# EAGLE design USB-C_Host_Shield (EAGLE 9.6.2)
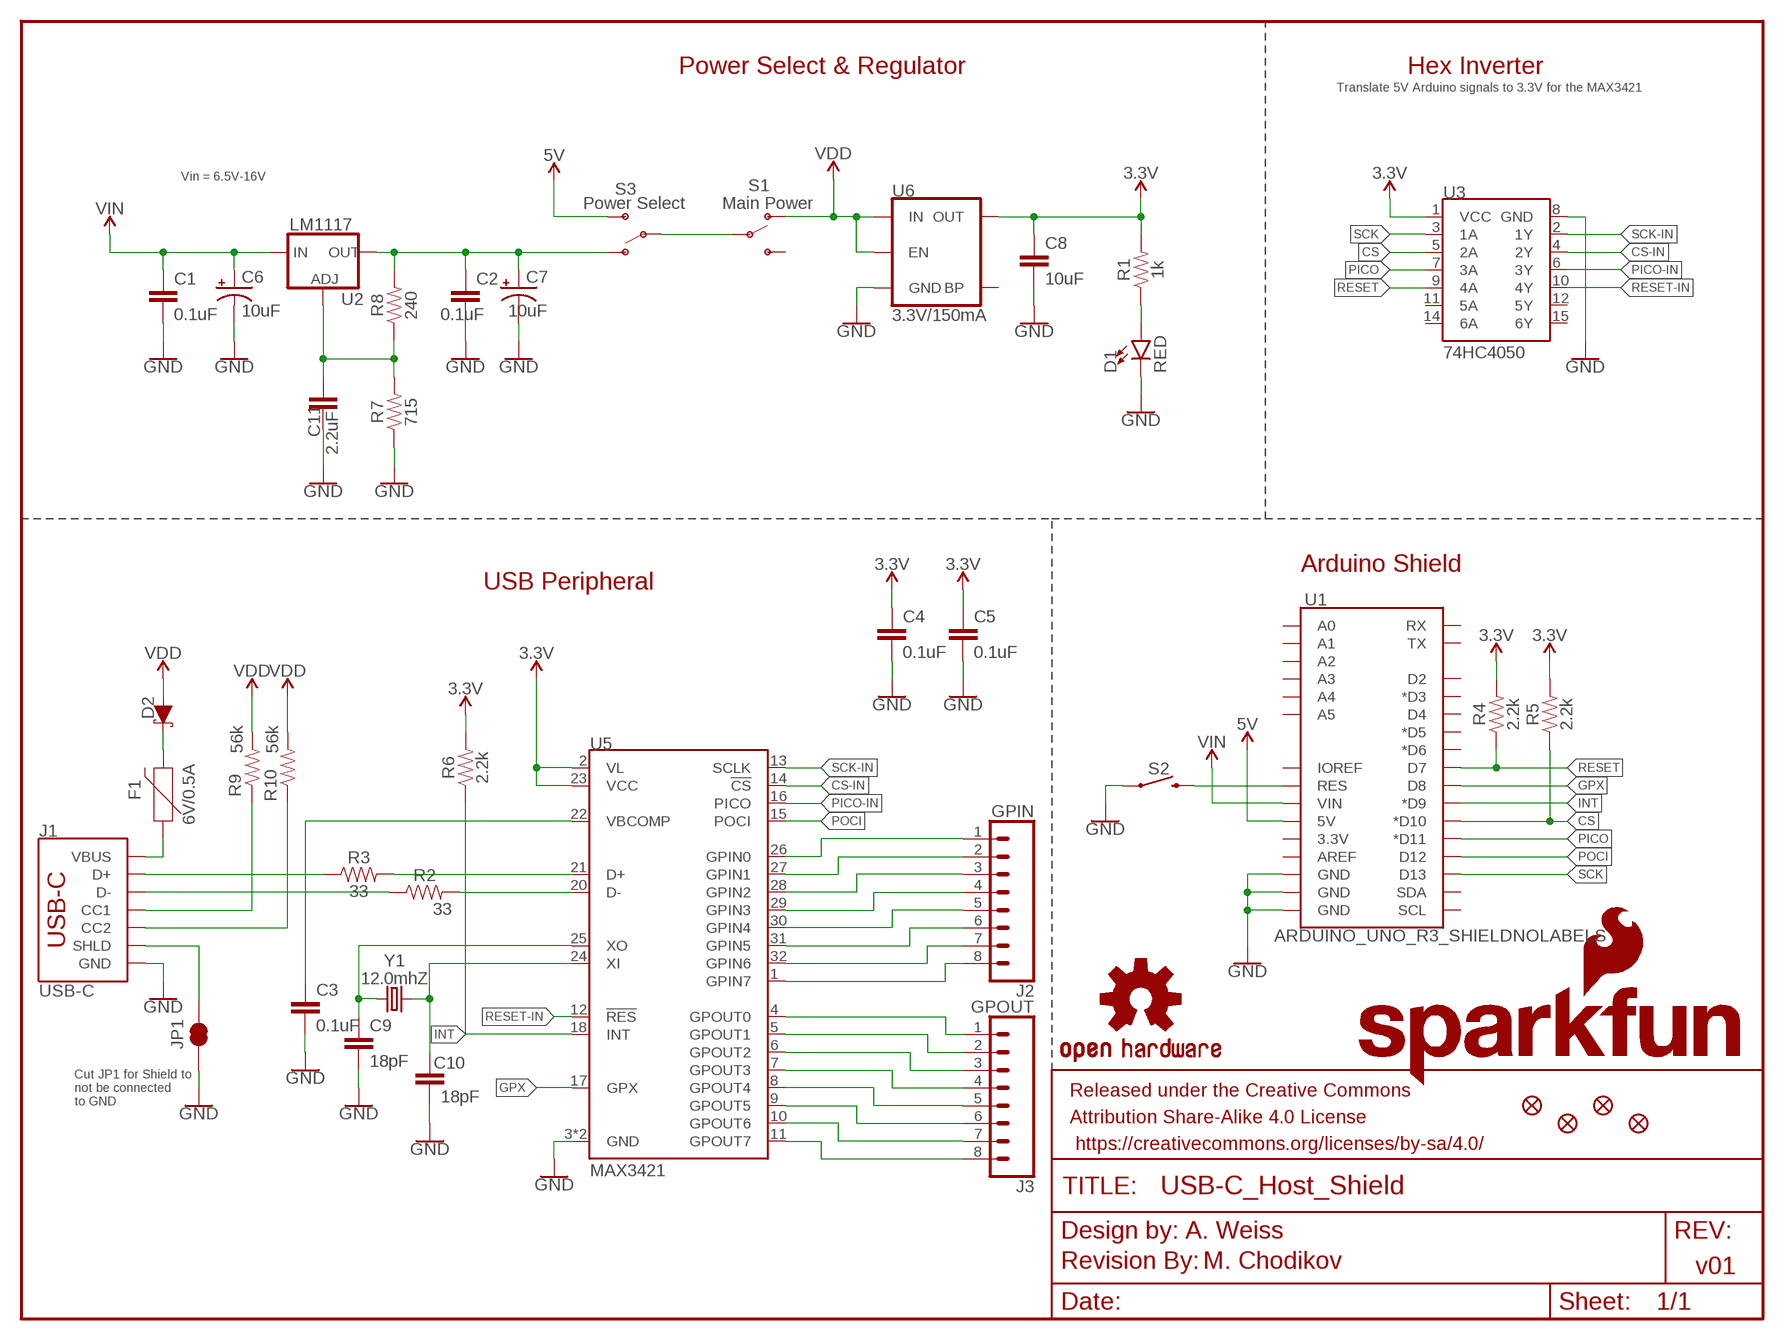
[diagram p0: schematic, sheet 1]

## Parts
C1  0.1uF  0.1UF-0603-25V-(+80/-20%)  [0603]
C2  0.1uF  0.1UF-0603-25V-(+80/-20%)  [0603]
C3  0.1uF  0.1UF-0603-25V-(+80/-20%)  [0603]
C4  0.1uF  0.1UF-0603-25V-(+80/-20%)  [0603]
C5  0.1uF  0.1UF-0603-25V-(+80/-20%)  [0603]
C6  10uF  10UF-POLAR-EIA3216-16V-10%(TANT)  [EIA3216]
C7  10uF  10UF-POLAR-EIA3216-16V-10%(TANT)  [EIA3216]
C8  10uF  10UF-0603-6.3V-20%  [0603]
C9  18pF  18PF-0603-50V-5%  [0603]
C10  18pF  18PF-0603-50V-5%  [0603]
C11  2.2uF  2.2UF-0603-10V-20%  [0603]
D1  RED  LED-RED0603  [LED-0603]
D2  1A/15V/220mV  DIODE-SCHOTTKY-LSM115JE3  [DO-214BA]
F1  6V/0.5A  PPTC_6V500MA-2  [1206]
FD1  FIDUCIALUFIDUCIAL  [FIDUCIAL-MICRO]
FD2  FIDUCIALUFIDUCIAL  [FIDUCIAL-MICRO]
FD3  FIDUCIALUFIDUCIAL  [FIDUCIAL-MICRO]
FD4  FIDUCIALUFIDUCIAL  [FIDUCIAL-MICRO]
FRAME1  FRAME-LETTER  [CREATIVE_COMMONS]
J1  USB-C  USB_C_2-LAYER_PADS  [USB-C-16P-2LAYER-PADS]
J2  GPIN  CONN_08"  [1X08]
J3  GPOUT  CONN_08"  [1X08]
JP1  JUMPER-SMT_2_NC_TRACE_SILK  [SMT-JUMPER_2_NC_TRACE_SILK]
LOGO1  OSHW-LOGOM  [OSHW-LOGO-M]
LOGO2  SFE_LOGO_NAME_FLAME.1_INCH  [SFE_LOGO_NAME_FLAME_.1]
LOGO3  SFE_LOGO_NAME_FLAME.2_INCH  [SFE_LOGO_NAME_FLAME_.2]
LOGO7  REVISION  [REVISION]
R1  1k  1KOHM-0603-1/10W-1%  [0603]
R2  33  33OHM-0603-1/10W-1%  [0603]
R3  33  33OHM-0603-1/10W-1%  [0603]
R4  2.2k  2.2KOHM-0603-1/10W-1%  [0603]
R5  2.2k  2.2KOHM-0603-1/10W-1%  [0603]
R6  2.2k  2.2KOHM-0603-1/10W-1%  [0603]
R7  715  715OHM-0603-1/10W-1%  [0603]
R8  240  240OHM-0603-1/10W-1%  [0603]
R9  56k  56KOHM  [0603]
R10  56k  56KOHM  [0603]
S1  Main Power  SWITCH-SPDT-SMD-AYZ0202  [SWITCH_DPDT_SMD_AYZ0202]
S2  MOMENTARY-SWITCH-SPST-SMD-5.2MM-TALL  [TACTILE_SWITCH_SMD_5.2MM]
S3  Power Select  SWITCH-SPDT-SMD-AYZ0202  [SWITCH_DPDT_SMD_AYZ0202]
U1  ARDUINO_UNO_R3_SHIELDNOLABELS  [UNO_R3_SHIELD_NOLABELS]
U2  LM1117  V_REG_LM1117SOT223  [SOT223]
U3  74HC4050  HEX_CONVERTER  [SO16]
U5  MAX3421  [TQFP32]
U6  3.3V/150mA  V_REG_MIC52053.3V  [SOT23-5]
Y1  12.0mhZ  CRYSTAL-12MHZ  [CRYSTAL-SMD-2X2.5MM]

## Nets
3.3V: C4.1 C5.1 C8.1 R1.2 R4.2 R5.2 R6.2 U3.1(VCC) U5.2(VL) U5.23(VCC) U6.5(OUT)
5V: S3.3(S) U1.5V
CC1: J1.A5(CC1) R9.1
CC2: J1.B5(CC2) R10.1
CS: R5.1 U1.D10(*D10) U3.5(2A)
CS-IN: U3.4(2Y) U5.14(!CS)
D_N [diff pairs]: J1.A7(D-) J1.B7(D-) R2.1
D_P [diff pairs]: J1.A6(D+) J1.B6(D+) R3.1
GND: C1.2 C2.2 C3.2 C4.2 C5.2 C6.- C7.- C8.2 C9.2 C10.2 C11.2 D1.C J1.GND J1.GND2(GND) JP1.1 R7.1 S2.1 U1.GND@0(GND) U1.GND@1(GND) U1.GND@2(GND) U3.8(GND) U5.3(GND) U5.19(GND) U6.2(GND)
GPIN0: J2.1 U5.26(GPIN0)
GPIN1: J2.2 U5.27(GPIN1)
GPIN2: J2.3 U5.28(GPIN2)
GPIN3: J2.4 U5.29(GPIN3)
GPIN4: J2.5 U5.30(GPIN4)
GPIN5: J2.6 U5.31(GPIN5)
GPIN6: J2.7 U5.32(GPIN6)
GPIN7: J2.8 U5.1(GPIN7)
GPOUT0: J3.1 U5.4(GPOUT0)
GPOUT1: J3.2 U5.5(GPOUT1)
GPOUT2: J3.3 U5.6(GPOUT2)
GPOUT3: J3.4 U5.7(GPOUT3)
GPOUT4: J3.5 U5.8(GPOUT4)
GPOUT5: J3.6 U5.9(GPOUT5)
GPOUT6: J3.7 U5.10(GPOUT6)
GPOUT7: J3.8 U5.11(GPOUT7)
GPX: U1.D8 U5.17(GPX)
INT: R6.1 U1.D9(*D9) U5.18(INT)
MAX_D_N: R2.2 U5.20(D-)
MAX_D_P: R3.2 U5.21(D+)
N$1: S2.3 U1.RES
N$2: S1.2(P) S3.2(P)
N$4: C11.1 R7.2 R8.1 U2.1(ADJ)
N$5: D2.C F1.2
N$6: C2.1 C7.+ R8.2 S3.1(O) U2.2(OUT) U2.4(OUT)
N$7: D1.A R1.1
N$8: J1.SHLD1(SHLD) J1.SHLD2(SHLD) J1.SHLD3(SHLD) J1.SHLD4(SHLD) JP1.2
PICO: U1.D11(*D11) U3.7(3A)
PICO-IN: U3.6(3Y) U5.16(PICO)
POCI: U1.D12 U5.15(POCI)
RESET: R4.1 U1.D7 U3.9(4A)
RESET-IN: U3.10(4Y) U5.12(!RES)
SCK: U1.D13 U3.3(1A)
SCK-IN: U3.2(1Y) U5.13(SCLK)
VBCOMP: C3.1 U5.22(VBCOMP)
VBUS: F1.1 J1.VBUS1(VBUS) J1.VBUS2(VBUS)
VDD: D2.A R9.2 R10.2 S1.1(O) U6.1(IN) U6.3(EN)
VIN: C1.1 C6.+ U1.VIN U2.3(IN)
XI: C10.1 U5.24(XI) Y1.P3
XO: C9.1 U5.25(XO) Y1.P1
Unconnected: S1.3(S) U1.3.3V U1.A0 U1.A1 U1.A2 U1.A3 U1.A4 U1.A5 U1.AREF U1.D2 U1.D3(*D3) U1.D4 U1.D5(*D5) U1.D6(*D6) U1.IOREF U1.RX U1.SCL U1.SDA U1.TX U3.11(5A) U3.12(5Y) U3.14(6A) U3.15(6Y) U6.4(BP)

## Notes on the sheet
- Power Select & Regulator | Hex Inverter
- Translate 5V Arduino signals to 3.3V for the MAX3421
- Vin = 6.5V-16V
- Arduino Shield
- USB Peripheral
- Cut JP1 for Shield to
  not be connected
  to GND
- A. Weiss
- M. Chodikov | v01

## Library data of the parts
C1-C5 = SparkFun-Capacitors:0.1UF: 0.1µF ceramic capacitors; PROD_ID: CAP-00810
C6 C7 = SparkFun-Capacitors:10UF-POLAR: 10.0µF polarized capacitors; PROD_ID: CAP-00811
C8 = SparkFun-Capacitors:10UF: 10.0µF ceramic capacitors; PROD_ID: CAP-11015
C9 C10 = SparkFun-Capacitors:18PF: 18pF ceramic capacitors; PROD_ID: CAP-08267
C11 = SparkFun-Capacitors:2.2UF: 2.2µF ceramic capacitors; PROD_ID: CAP-07888
D1 = SparkFun-LED:LED-RED: Red SMD LED; PROD_ID: DIO-00819
D2 = SparkFun-DiscreteSemi:DIODE-SCHOTTKY: Schottky diode; PROD_ID: DIO-15217
F1 = SparkFun-Fuses:PPTC: Resettable Fuse PPTC; PROD_ID: RES-08585
FD1-FD4 = SparkFun-Aesthetics:FIDUCIAL: Fiducial Alignment Points
FRAME1 = SparkFun-Aesthetics:FRAME-LETTER: Schematic Frame - Letter
J1 = SparkFun-Connectors:USB_C: USB Type C 16Pin Connector Super Speed pins not available on the 16-pin purely SMD connector so this part is best for USB 2.0 implementations. D1 and D2 are tied together enabling D+/- no matter which way the cable is plugged into the connector. The two channel configuration pins (CC1/2) are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; PROD_ID: CONN-14122
J2 J3 = SparkFun-Connectors:CONN_08: Multi connection point. Often used as Generic Header-pin footprint for 0.1 inch spaced/style header connections On any of the 0.1 inch spaced packages, you can populate with these: Break Away Headers - Straight (PRT-00116) Break Away Male Headers - Right Angle (PRT-00553) Female Headers (PRT-00115)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; PROD_ID: CONN-08438
JP1 = SparkFun-Jumpers:JUMPER-SMT_2_NC_TRACE: Normally closed trace jumper
LOGO1 = SparkFun-Aesthetics:OSHW-LOGO: Open-Source Hardware (OSHW) Logo
LOGO2 LOGO3 = SparkFun-Aesthetics:SFE_LOGO_NAME_FLAME: SparkFun Font Logo w/ Flame
LOGO7 = SparkFun-Aesthetics:REVISION: "Revision By" Text
R1 = SparkFun-Resistors:1KOHM: 1kΩ resistor; PROD_ID: RES-07856
R2 R3 = SparkFun-Resistors:33OHM: 33Ω resistor; PROD_ID: RES-08270
R4-R6 = SparkFun-Resistors:2.2KOHM: 2.2kΩ resistor; PROD_ID: RES-08272
R7 = SparkFun-Resistors:715OHM: 715Ω resistor; PROD_ID: RES-07850
R8 = SparkFun-Resistors:240OHM: 240Ω resistor; PROD_ID: RES-07849
R9 R10 = SparkFun-Resistors:56KOHM: 56kΩ Resistor; PROD_ID: RES-17211
S1 S3 = SparkFun-Switches:SWITCH-SPDT: Single Pole, Double Throw (SPDT) Switch Single-pole, double-throw (SPDT) switch. Variant Overview SMD-AYZ0202 Surface Mount DPDT Switch (COM-00597) Used on e.g. LilyPad Arduino USB - ATmega32U4 Board PTH-11.6X4.0MM SPDT Mini Power Switch (COM-00102) Used on e.g. SparkFun Simon Says - Through-Hole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; PROD_ID: SWCH-08179; SF_ID: COM-00597
S2 = SparkFun-Switches:MOMENTARY-SWITCH-SPST: Momentary Switch (Pushbutton) - SPST; PROD_ID: SWCH-14139
U1 = SparkFun-Boards:ARDUINO_UNO_R3_SHIELD: Arduino R3 Shield Footprint Shield form compatible with the Arduino Uno R3. SparkFun Products: MG2639 Cellular Shield MIDI Shield R3 Stackable Headers Kit
U2 = SparkFun-IC-Power:V_REG_LM1117: Voltage Regulator LM1117 Standard adjustable voltage regulator but in SMD form. Spark Fun Electronics SKU : COM-00595; PROD_ID: VREG-08170
U3 = SparkFun-IC-Comms:HEX_CONVERTER: 74HC4050 Hex Buffer 74HC4050 Hex Buffer Level Shifter SMD SO016 SparkFun Products CAN-BUS Shield (DEV-13262) SparkFun MP3 Player Shield (DEV-12660) SparkFun microSD Shield (DEV-12761) SparkFun USB Host Shield (DEV-09947); PROD_ID: IC-09604
U5 = SparkFun-IC-Microcontroller:MAX3421: USB Peripheral/Host Controller with SPI Interface; PROD_ID: IC-09517
U6 = SparkFun-IC-Power:V_REG_MIC5205: V_REG MIC5205 Standard 3.3V, 5V, and Adjustable 150mA LDO voltage regulator in SOT-23 layout. Micrel part MIC5205. BP (by-pass) pin is used to lower output noise with 470pF cap, may be left open. On the adjustable version BP is used to set output.; PROD_ID: VREG-00822
Y1 = SparkFun-Clocks:CRYSTAL-12MHZ: 12.0MHz Crystal; PROD_ID: XTAL-15540

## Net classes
2 diff pairs: width 0.089 mm

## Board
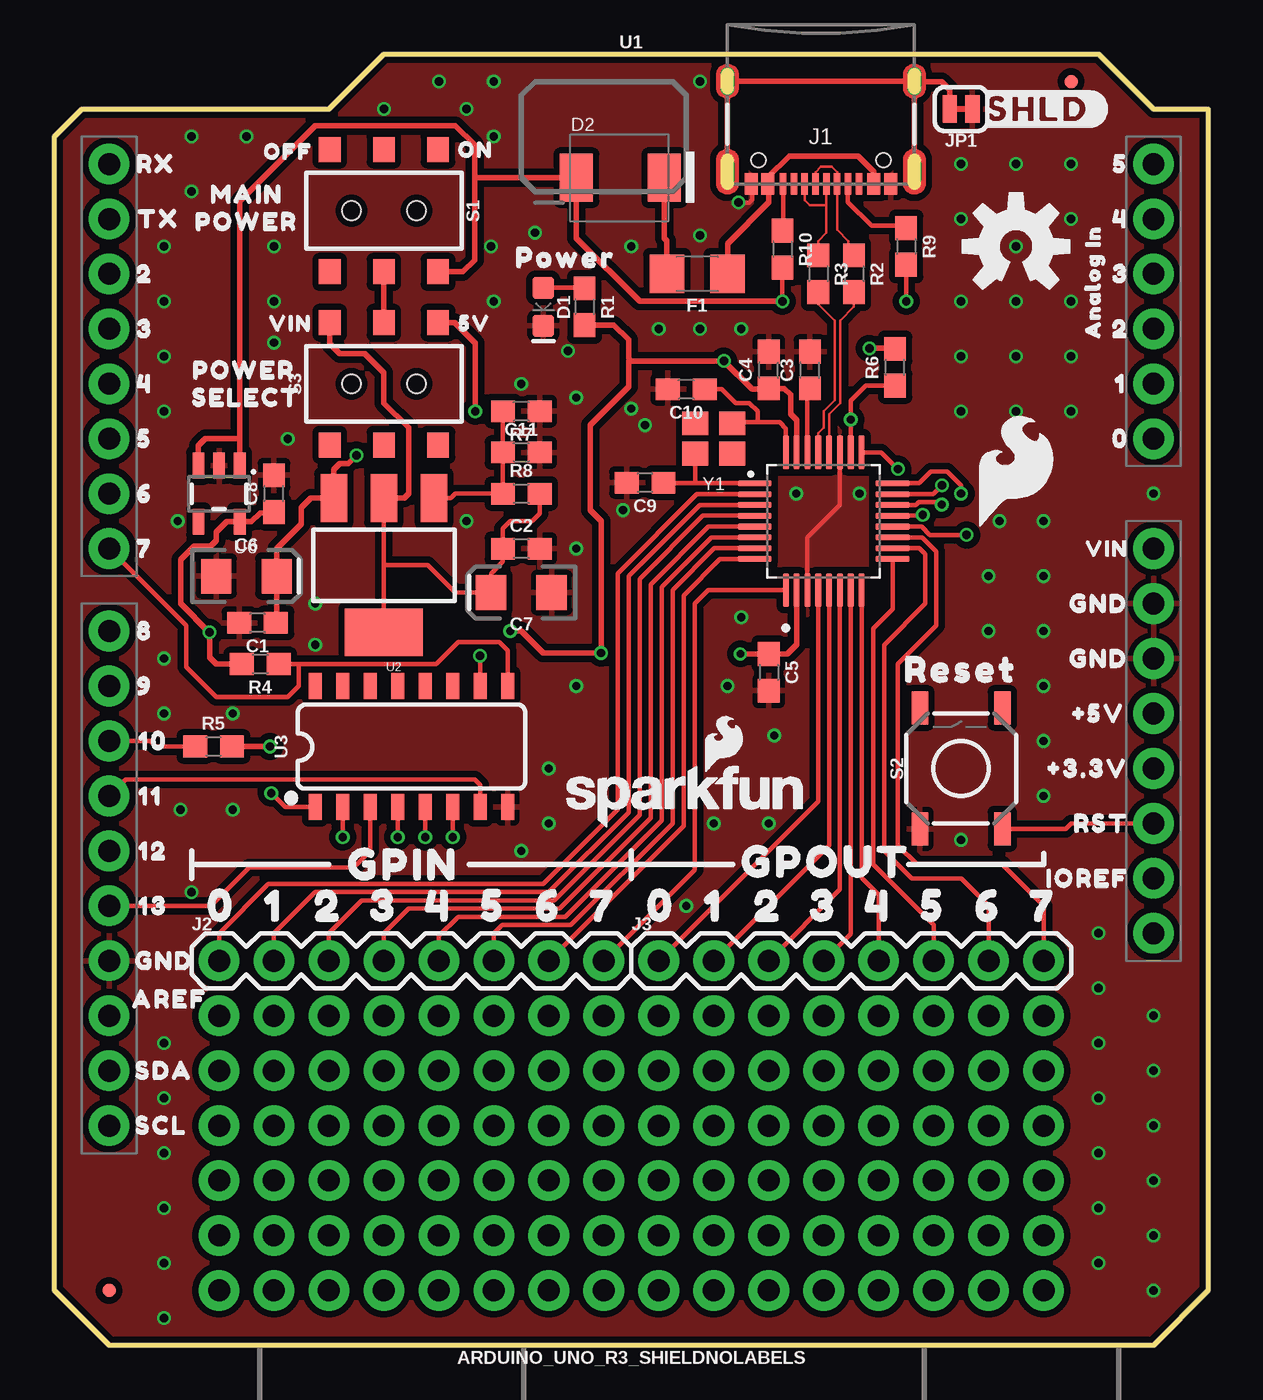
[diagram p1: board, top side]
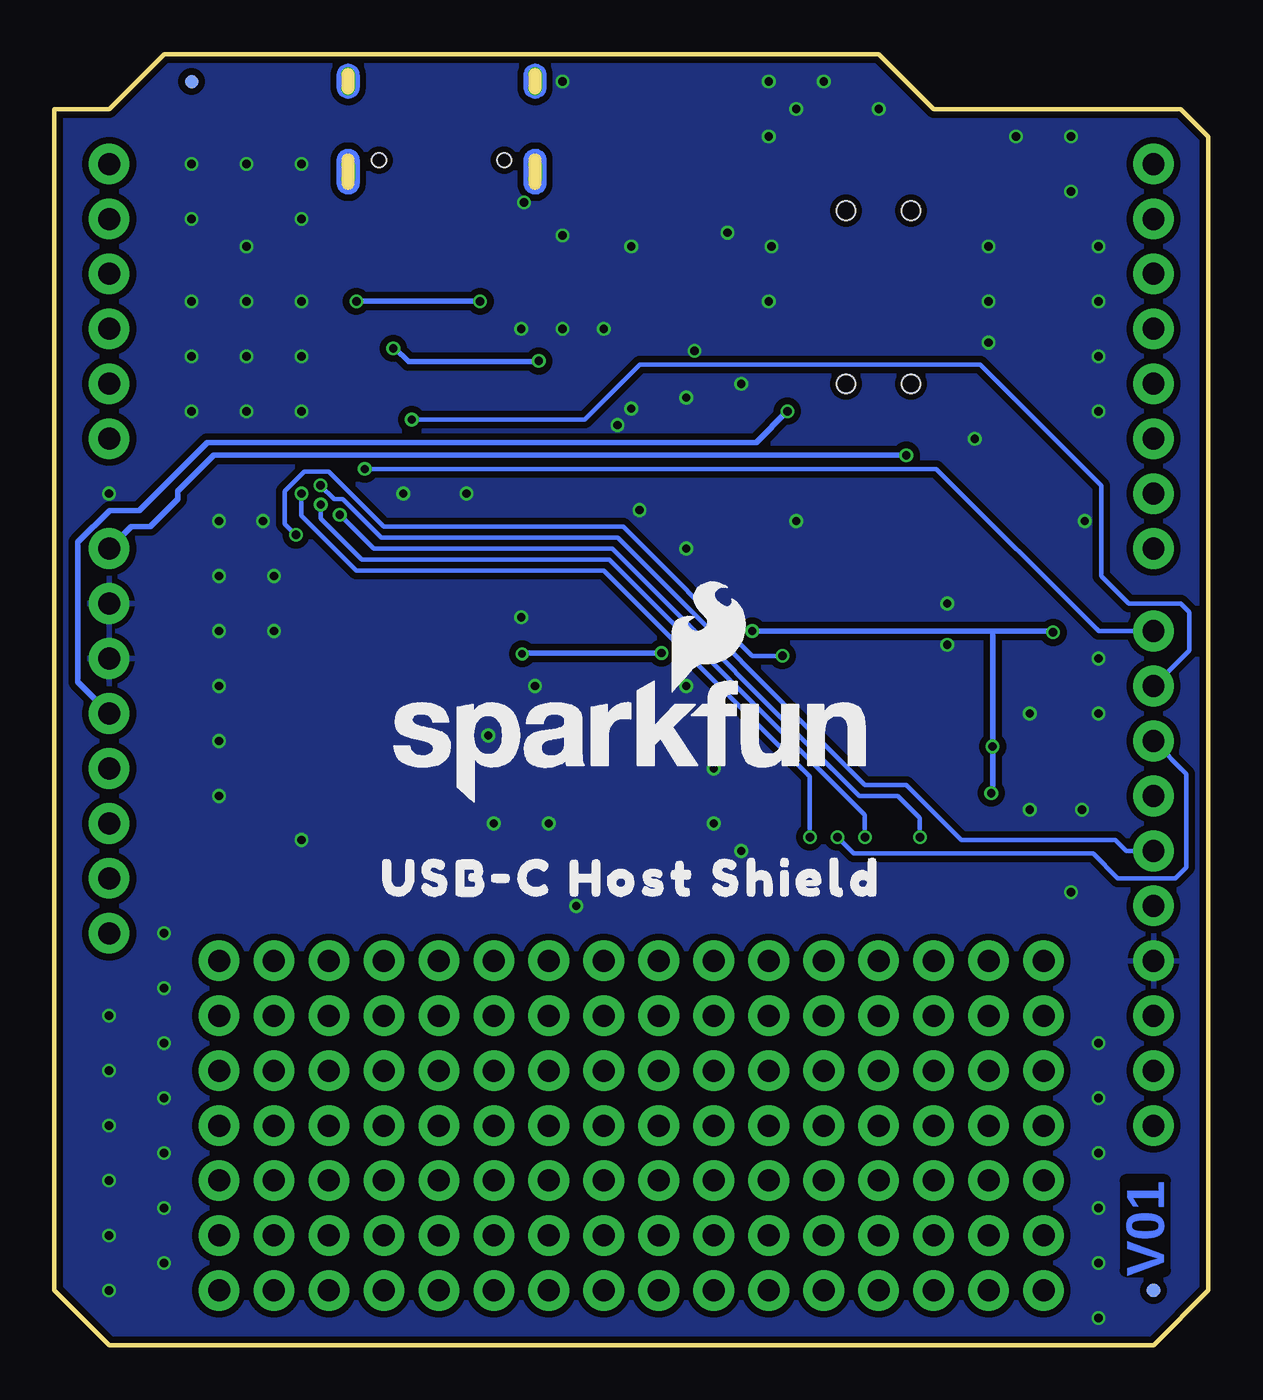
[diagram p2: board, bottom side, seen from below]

Size 53.34 x 59.69 mm. Coordinates in mm from the lower left corner, seen from the top.
Outline: 2.54,0 50.8,0 53.34,2.54 53.34,57.15 50.8,57.15 48.26,59.69 15.24,59.69 12.7,57.15 1.27,57.15 0,55.88 0,2.54 2.54,0
Copper layers (1*16): Top 0.035mm / dielectric 1.5mm / Bottom 0.035mm
Design rules "SparkFun-2-Layer-Minimum-JLCPCB *": minimum track width 5mil, minimum drill 0.3mm, track to track 5mil, track to pad 5mil, pad to pad 5mil, via to via 5mil, smd to smd 5mil, copper to edge 7mil, drill to drill 7mil, minimum pad ring 5mil, minimum via ring 5mil, stop-mask expansion 2.5mil, vias tented up to drill 25mil, thermal gap 10mil

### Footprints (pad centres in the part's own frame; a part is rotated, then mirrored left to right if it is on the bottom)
0603 = smd 1.1 x 1: 1 -0.85,0; 2 0.85,0
EIA3216 = smd 1.4 x 1.6: + 1.4,0; - -1.4,0
LED-0603 = smd 1 x 1: A -0.877,0; C 0.877,0
DO-214BA = smd 1.52 x 2.21: A -2.032,0; C 2.038,0
1206 = smd 1.6 x 1.8: 1 -1.4,0; 2 1.4,0
FIDUCIAL-MICRO = smd 0.635 x 0.635: 1 0,0
USB-C-16P-2LAYER-PADS = smd 0.3 x 1: A5 -1.25,-0.34; A6 -0.25,-0.34; A7 0.25,-0.34; A8 1.25,-0.34; B5 1.75,-0.34; B6 0.75,-0.34; B7 -0.75,-0.34; B8 -1.75,-0.34 | smd 0.6 x 1: GND -3.225,-0.34; GND2 3.225,-0.34; VBUS1 -2.45,-0.34; VBUS2 2.45,-0.34 | drill 0.4 pad 0.6 long: SHLD1 -4.318,-0.915; SHLD2 4.318,-0.915; SHLD3 -4.318,-5.095; SHLD4 4.318,-5.095 | hole 0.65: -2.89,-1.445; 2.89,-1.445
1X08 = drill 1.016 pad 1.88: 1 0,0; 2 2.54,0; 3 5.08,0; 4 7.62,0; 5 10.16,0; 6 12.7,0; 7 15.24,0; 8 17.78,0
SMT-JUMPER_2_NC_TRACE_SILK = smd 0.66 x 1.27: 1 -0.521,0; 2 0.521,0
SWITCH_DPDT_SMD_AYZ0202 = smd 1 x 1.15: 1 -2.5,2.825; 2 0,2.825; 3 2.5,2.825; 4 -2.5,-2.825; 5 0,-2.825; 6 2.5,-2.825 | hole 0.85: 1.5,0; -1.5,0
TACTILE_SWITCH_SMD_5.2MM = smd 1.524 x 0.762: 1 -2.794,1.905; 2 2.794,1.905; 3 -2.794,-1.905; 4 2.794,-1.905
UNO_R3_SHIELD_NOLABELS = drill 1.016 pad 1.88: 3.3V 24.13,-3.81; 5V 24.13,-1.27; A0 24.13,11.43; A1 24.13,13.97; A2 24.13,16.51; A3 24.13,19.05; A4 24.13,21.59; A5 24.13,24.13; AREF -24.13,-15.24; D2 -24.13,19.05; D3 -24.13,16.51; D4 -24.13,13.97; D5 -24.13,11.43; D6 -24.13,8.89; D7 -24.13,6.35; D8 -24.13,2.54; D9 -24.13,0; D10 -24.13,-2.54; D11 -24.13,-5.08; D12 -24.13,-7.62; D13 -24.13,-10.16; GND@0 24.13,1.27; GND@1 24.13,3.81; GND@2 -24.13,-12.7; IOREF 24.13,-8.89; NC 24.13,-11.43; RES 24.13,-6.35; RX -24.13,24.13; SCL -24.13,-20.32; SDA -24.13,-17.78; TX -24.13,21.59; VIN 24.13,6.35
SOT223 = smd 1.219 x 2.235: 1 -2.311,-3.099; 2 0,-3.099; 3 2.311,-3.099 | smd 3.6 x 2.2: 4 0,3.099
SO16 = smd 0.6 x 1.2: 1 -4.445,-2.8; 2 -3.175,-2.8; 3 -1.905,-2.8; 4 -0.635,-2.8; 5 0.635,-2.8; 6 1.905,-2.8; 7 3.175,-2.8; 8 4.445,-2.8; 9 4.445,2.8; 10 3.175,2.8; 11 1.905,2.8; 12 0.635,2.8; 13 -0.635,2.8; 14 -1.905,2.8; 15 -3.175,2.8; 16 -4.445,2.8
TQFP32 = smd 1.56 x 0.28: 1 -3.18,1.75; 2 -3.18,1.25; 3 -3.18,0.75; 4 -3.18,0.25; 5 -3.18,-0.25; 6 -3.18,-0.75; 7 -3.18,-1.25; 8 -3.18,-1.75; 17 3.18,-1.75; 18 3.18,-1.25; 19 3.18,-0.75; 20 3.18,-0.25; 21 3.18,0.25; 22 3.18,0.75; 23 3.18,1.25; 24 3.18,1.75 | smd 0.28 x 1.56: 9 -1.75,-3.18; 10 -1.25,-3.18; 11 -0.75,-3.18; 12 -0.25,-3.18; 13 0.25,-3.18; 14 0.75,-3.18; 15 1.25,-3.18; 16 1.75,-3.18; 25 1.75,3.18; 26 1.25,3.18; 27 0.75,3.18; 28 0.25,3.18; 29 -0.25,3.18; 30 -0.75,3.18; 31 -1.25,3.18; 32 -1.75,3.18
SOT23-5 = smd 0.55 x 1.2: 1 -0.95,-1.3; 2 0,-1.3; 3 0.95,-1.3; 4 0.95,1.3; 5 -0.95,1.3
CRYSTAL-SMD-2X2.5MM = smd 1.2 x 1.1: P1 0.846,0.69; P2 -0.854,0.69; P3 -0.854,-0.71; P4 0.846,-0.71

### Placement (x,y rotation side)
C1  9.4,33.4 180 top
C2  21.59,36.83 0 top
C3  34.92,45.09 90 top
C4  33.02,45.09 90 top
C5  33.02,31.11 270 top
C6  8.89,35.56 0 top
C7  21.59,34.8 180 top
C8  10.16,39.37 90 top
C9  27.3,39.88 180 top
C10  29.21,44.2 180 top
C11  21.59,41.27 0 top
D1  22.61,48.01 270 top
D2  26.16,53.98 0 top
F1  29.72,49.53 180 top
FD1  2.54,2.54 0 bottom
FD2  2.54,2.54 90 top
FD3  46.99,58.42 0 bottom
FD4  46.99,58.42 0 top
FRAME1  not placed on the board
J1  35.43,53.34 180 top
J2  7.62,17.78 0 top
J3  27.94,17.78 0 top
JP1  41.91,57.15 180 top
LOGO1  44.45,50.8 0 top
LOGO2  29.21,25.4 0 top
LOGO3  26.67,27.94 0 bottom
LOGO7  not placed on the board
R1  24.51,48.01 270 top
R2  36.96,49.53 270 top
R3  35.31,49.53 270 top
R4  9.53,31.5 180 top
R5  7.37,27.69 0 top
R6  38.86,45.21 90 top
R7  21.59,43.18 180 top
R8  21.59,39.37 0 top
R9  39.37,50.8 270 top
R10  33.66,50.67 270 top
S1  15.24,52.45 180 top
S2  41.91,26.67 90 top
S3  15.24,44.45 0 top
U1  26.67,30.48 0 top
U2  15.24,36.07 180 top
U3  16.51,27.69 0 top
U5  35.56,38.1 90 top
U6  7.62,39.37 180 top
U$1  [5V6]  19.43,47.24 0 top
U$2  [POWER23]  23.62,50.29 0 top
U$3  [GPIN42]  16.13,22.22 0 top
U$4  [SFE_LOGO_FLAME_.2]  44.45,40.39 0 top
U$5  [ON26]  19.47,55.27 0 top
U$6  [RESET25]  41.91,31.24 0 top
U$7  [OFF27]  10.82,55.18 0 top
U$8  [ANALOG_IN28]  48.01,49.15 90 top
U$9  [USB#C_HOST_SHIELD32]  26.67,21.59 0 bottom
U$10  [POWER11]  8.76,45.09 0 top
U$11  [SHLD#33]  45.47,57.15 0 top
U$12  [VIN7]  10.92,47.24 0 top
U$13  [SELECT12]  8.89,43.81 0 top
U$14  [POWER38]  8.89,51.94 0 top
U$15  [MAIN40]  8.89,53.21 0 top
U$16  [GPOUT44]  35.69,22.35 0 top
U$17  [045]  28.07,20.32 0 top
U$18  [146]  30.48,20.32 0 top
U$19  [2147]  33.02,20.32 0 top
U$20  [32148]  35.56,20.32 0 top
U$21  [4332150]  38.1,20.32 0 top
U$22  [4332150]  17.78,20.32 0 top
U$23  [54332151]  20.32,20.32 0 top
U$24  [654332152]  43.18,20.32 0 top
U$25  [54332151]  40.64,20.32 0 top
U$26  [654332152]  22.86,20.32 0 top
U$27  [7654332153]  45.72,20.32 0 top
U$28  [7654332153]  25.4,20.32 0 top
U$29  [045]  7.75,20.32 0 top
U$30  [146]  10.16,20.32 0 top
U$31  [2147]  12.7,20.32 0 top
U$32  [32148]  15.24,20.32 0 top
U$33  [#3#3V131211211109876543234]  47.75,26.67 0 top
U$34  [#5V131211211109876543234]  48.26,29.21 0 top
U$35  [GND131211211109876543229]  48.26,31.75 0 top
U$36  [GND131211211109876543229]  48.26,34.29 0 top
U$37  [GND131211211109876543229]  5.08,17.78 0 top
U$38  [RX14]  4.7,54.61 0 top
U$39  [TX15]  4.83,52.07 0 top
U$40  [216]  4.19,49.53 0 top
U$41  [3217]  4.19,46.99 0 top
U$42  [43218]  4.19,44.45 0 top
U$43  [543219]  4.19,41.91 0 top
U$44  [6543220]  4.19,39.37 0 top
U$45  [76543221]  4.19,36.83 0 top
U$46  [876543222]  4.19,33.02 0 top
U$47  [9876543223]  4.19,30.48 0 top
U$48  [109876543224]  4.57,27.94 0 top
U$49  [11109876543225]  4.45,25.4 0 top
U$50  [1211211109876543227]  4.57,22.86 0 top
U$51  [131211211109876543228]  4.57,20.32 0 top
U$52  [AREF131211211109876543230]  5.33,16 0 top
U$53  [SDA131211211109876543231]  5.08,12.7 0 top
U$54  [SCL131211211109876543232]  4.95,10.16 0 top
U$55  [0131211211109876543236]  49.28,41.91 0 top
U$56  [1131211211109876543239]  49.28,44.45 0 top
U$57  [216]  49.28,46.99 0 top
U$58  [3217]  49.28,49.53 0 top
U$59  [43218]  49.28,52.07 0 top
U$60  [543219]  49.28,54.61 0 top
U$61  [VIN7]  48.64,36.83 0 top
U$62  [RST131211211109876543234]  48.39,24.13 0 top
U$63  [IOREF131211211109876543235]  47.75,21.59 0 top
Y1  30.48,41.91 180 top

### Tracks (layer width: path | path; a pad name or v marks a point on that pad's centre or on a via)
3.3V  (via drill 0.35, 0.38)
  Top 0.203: v7.17,32.96 v7.18,32.96 | v10.03,25.53 10.67,24.89 U3.1 | C4.1 33.06,44.23
  Top 0.254: C8.1 10.16,38.48 9.53,38.48 9.11,38.07 U6.5 7.97,38.07 7.49,37.59 7.49,37.21 7.24,36.96 6.48,36.96 5.84,36.32 5.84,34.29 v7.17,32.96 | 26.67,45.51 26.54,45.51 26.54,44.32 24.77,42.55 24.77,38.61 25.27,38.1 v25.27,32 22.61,32 21.59,33.02 v21.08,33.02 | 26.67,45.51 v30.95,45.51 32.26,44.2 33.02,44.2 33.06,44.23 33.74,44.23 34.04,43.94 34.04,43.05 34.31,42.78 U5.23 | 26.67,45.51 26.54,45.63 26.54,46.48 25.87,47.16 R1.2 | v37.67,46.09 38.84,46.09 R6.2 | v31.71,31.96 C5.1 33.87,31.96 34.31,32.41 U5.2 | v7.18,32.96 7.18,31.81 7.49,31.5 R4.2 | R5.2 v9.97,27.69
  Bottom 0.203: 9.97,25.59 v10.03,25.53
  Bottom 0.254: v37.67,46.09 v37.66,46.1 37.59,46.1 36.96,45.47 30.99,45.47 v30.95,45.51 | v25.27,32 31.67,32 v31.71,31.96 | v7.18,32.96 7.24,33.02 10.03,33.02 | 10.03,33.02 v21.08,33.02 | 10.03,33.02 9.97,32.96 v9.97,27.69 9.97,25.59
5V  (via drill 0.38)
  Top 0.254: v19.46,43.18 19.46,46.33 18.51,47.27 S3.3
  Bottom 0.254: v19.46,43.18 20.89,41.74 46.26,41.74 49.4,38.6 50.77,38.6 52.25,37.12 52.25,30.66 U1.5V
CC1
  Top 0.203: J1.A5 36.68,52.85 37.78,51.75 39.27,51.75 R9.1
CC2
  Top 0.203: J1.B5 33.68,51.55 R10.1
CS  (via drill 0.38)
  Top 0.203: U3.5 v17.14,23.49 | R5.1 4.7,27.69 4.45,27.94 U1.D10
  Bottom 0.203: v17.14,23.49 16.38,22.73 5.33,22.73 4.19,21.59 1.52,21.59 1.02,22.1 1.02,26.42 U1.D10
CS-IN  (via drill 0.38)
  Top 0.203: v41.02,38.86 40.89,38.99 39.96,38.99 39.82,38.85 U5.14 | U3.4 v15.88,23.49
  Bottom 0.203: v41.02,38.86 41.02,38.23 39.12,36.32 27.69,36.32 15.88,24.51 v15.88,23.49
D_N
  Top 0.127: R2.1 36.68,50.65 36.7,50.67 36.7,51.05 36.18,51.57 J1.B7 36.18,54.24 35.94,54.48 35.43,54.48 35.18,54.23 J1.A7
D_P
  Top 0.127: J1.A6 35.68,52.7 | 35.68,52.7 35.68,51.43 35.31,51.05 R3.1 | 35.68,52.7 34.92,52.7 34.68,52.95 J1.B6
GND  (via drill 0.38)
  Top 0.203: v31.62,52.83 32.13,52.83 32.26,52.96 32.26,53.63 J1.GND2 | U5.19 36.31,38.85 34.81,37.35 U5.3
  other vias: 6.35,20.95 5.08,1.27 5.08,6.35 5.08,3.81 46.99,54.61 44.45,54.61 46.99,52.07 44.45,50.8 17.78,58.42 50.8,15.24 50.8,12.7 50.8,10.16 50.8,5.08 26.67,43.31 24.13,43.81 27.3,42.55 41.91,54.61 15.24,57.15 5.08,8.89 5.08,11.43 50.8,7.62 48.26,6.35 48.26,8.89 48.26,11.43 48.26,13.97 48.26,16.51 50.8,39.37 48.26,3.81 50.8,2.54 5.08,13.97 19.05,57.15 45.72,27.94 12.06,32.38 5.08,31.75 22.23,51.44 26.67,50.8 27.94,46.99 31.75,46.99 29.84,46.99 34.29,39.37 37.21,39.37 12.06,34.29 19.05,38.1 24.13,36.83 24.13,30.48 22.86,26.67 22.86,24.13 21.59,22.86 8.26,24.77 5.84,24.77 5.08,29.21 5.08,45.72 5.08,43.18 6.35,53.34 6.35,55.88 8.89,55.88 41.91,48.26 44.45,48.26 46.99,48.26 41.91,45.72 44.45,45.72 46.99,45.72 41.91,43.18 44.45,43.18 46.99,43.18 45.72,38.1 45.72,35.56 43.18,35.56 45.72,33.02 43.18,33.02 45.72,30.48 20.32,58.42 5.08,50.8 5.71,38.1 10.79,41.91 10.16,46.35 5.08,48.26 10.16,48.26 20.19,50.8 20.32,48.26 23.75,45.97 21.59,44.45 26.29,38.61 31.11,30.48 31.75,33.66 33.02,24.13 30.48,24.13 29.21,20.32 48.26,19.05 45.72,25.4 41.91,23.37 8.26,29.21 29.84,58.42 29.84,51.31 20.32,55.88 43.69,38.1 10.16,50.8 33.27,28.19 41.91,52.07
  pour Top (isolate 0.305): 1.27,57.15 12.7,57.15 15.24,59.69 48.26,59.69 50.8,57.15 53.34,57.15 53.34,2.54 50.8,0 2.54,0 0,2.54 0,55.88
  pour Bottom (isolate 0.305): 0,2.54 0,55.88 1.27,57.15 12.7,57.15 15.24,59.69 48.26,59.69 50.8,57.15 53.34,57.15 53.34,2.54 50.8,0 2.54,0
GPIN0
  Top 0.203: J2.1 7.62,19.05 9.91,21.34 22.61,21.34 26.04,24.77 26.04,35.69 29.7,39.35 U5.26
GPIN1
  Top 0.203: J2.2 10.16,19.05 12.06,20.95 22.86,20.95 26.54,24.64 26.54,35.56 29.83,38.85 U5.27
GPIN2
  Top 0.203: J2.3 12.7,19.05 14.22,20.57 23.11,20.57 27.05,24.51 27.05,35.43 29.97,38.35 U5.28
GPIN3
  Top 0.203: J2.4 15.24,19.05 16.38,20.19 23.37,20.19 27.56,24.38 27.56,35.18 30.23,37.85 U5.29
GPIN4
  Top 0.203: J2.5 17.78,18.92 18.67,19.81 23.62,19.81 28.07,24.26 28.07,35.05 30.36,37.35 U5.30
GPIN5
  Top 0.203: J2.6 20.32,19.05 20.7,19.43 23.88,19.43 28.57,24.13 28.57,34.92 30.5,36.85 U5.31
GPIN6
  Top 0.203: J2.7 29.08,24 29.08,34.67 30.76,36.35 U5.32
GPIN7
  Top 0.203: J2.8 29.59,21.97 29.59,34.29 30.22,34.92 U5.1
GPOUT0
  Top 0.203: J3.1 35.31,25.15 U5.4
GPOUT1
  Top 0.203: J3.2 35.81,23.11 U5.5
GPOUT2
  Top 0.203: J3.3 36.31,21.07 U5.6
GPOUT3
  Top 0.203: J3.4 36.81,19.03 U5.7
GPOUT4
  Top 0.203: J3.5 38.1,20.83 37.31,21.62 U5.8
GPOUT5
  Top 0.203: J3.6 40.64,19.43 37.85,22.22 37.85,33.15 38.74,34.04 U5.9
GPOUT6
  Top 0.203: J3.7 43.18,20.32 41.91,21.59 39.62,21.59 38.35,22.86 38.35,32.38 40.26,34.29 40.26,36.58 39.98,36.85 U5.10
GPOUT7
  Top 0.203: J3.8 45.72,20.32 43.81,22.22 39.88,22.22 38.99,23.11 38.99,31.5 40.77,33.27 40.77,36.7 40.12,37.35 U5.11
GPX  (via drill 0.38)
  Top 0.203: v38.99,40.51 38.22,41.28 U5.17
  Bottom 0.203: v38.99,40.51 12.57,40.51 5.08,33.02 U1.D8
INT  (via drill 0.38)
  Top 0.203: R6.1 37.5,44.36 36.81,43.67 v36.81,42.8 U5.18
  Bottom 0.203: v36.81,42.8 28.83,42.8 26.29,45.34 10.54,45.34 4.95,39.75 4.95,35.56 3.68,34.29 1.27,34.29 0.89,33.91 0.89,32.13 U1.D9
MAX_D_N
  Top 0.127: R2.2 36.96,48.01 36.32,47.37 36.32,43.56 35.81,43.05 U5.20
MAX_D_P
  Top 0.127: R3.2 35.31,48.13 36.07,47.37 36.07,43.69 35.56,43.18 35.56,43.16 35.56,43.15 35.56,42.41 35.31,42.16 U5.21
N$1
  Top 0.203: S2.3 46.74,23.88 46.99,24.13 U1.RES
N$2
  Top 0.254: S3.2 S1.2
N$3  (via drill 1.02 pad 1.88)
  other vias: 7.62,2.54
N$4
  Top 0.203: R7.2 C11.1 R8.1 18.54,39.37 18.34,39.17 U2.1
N$5
  Top 0.254: F1.2 28.32,51.06 28.19,51.18 D2.C
N$6
  Top 0.203: R8.2 22.44,38.44 22.1,38.1 21.08,38.1 20.74,37.76 C2.1 20.74,36.23 20.19,35.68 C7.+ 18.54,34.8 17.27,36.07 15.24,36.07 | U2.2 15.24,36.07 | 15.24,36.07 U2.4
  Top 0.254: U2.2 16.18,39.17 16.38,39.37 16.38,42.42 15.24,43.56 15.24,44.96 14.35,45.85 13.21,45.85 12.74,46.31 S3.1
N$7
  Top 0.203: D1.A 24.48,48.88 R1.1
N$8
  Top 0.254: J1.SHLD3 J1.SHLD4 J1.SHLD2 | J1.SHLD3 J1.SHLD1 | JP1.2 41.39,58.04 41.01,58.42 39.77,58.42 J1.SHLD3
N$32  (via drill 1.02 pad 1.88)
  other vias: 7.62,15.24
N$33  (via drill 1.02 pad 1.88)
  other vias: 10.16,15.24
N$35  (via drill 1.02 pad 1.88)
  other vias: 12.7,15.24
N$38  (via drill 1.02 pad 1.88)
  other vias: 15.24,15.24
N$39  (via drill 1.02 pad 1.88)
  other vias: 17.78,15.24
N$40  (via drill 1.02 pad 1.88)
  other vias: 20.32,15.24
N$41  (via drill 1.02 pad 1.88)
  other vias: 22.86,15.24
N$42  (via drill 1.02 pad 1.88)
  other vias: 25.4,15.24
N$43  (via drill 1.02 pad 1.88)
  other vias: 27.94,15.24
N$44  (via drill 1.02 pad 1.88)
  other vias: 30.48,15.24
N$45  (via drill 1.02 pad 1.88)
  other vias: 33.02,15.24
N$46  (via drill 1.02 pad 1.88)
  other vias: 35.56,15.24
N$47  (via drill 1.02 pad 1.88)
  other vias: 38.1,15.24
N$48  (via drill 1.02 pad 1.88)
  other vias: 40.64,15.24
N$49  (via drill 1.02 pad 1.88)
  other vias: 43.18,15.24
N$50  (via drill 1.02 pad 1.88)
  other vias: 45.72,15.24
N$51  (via drill 1.02 pad 1.88)
  other vias: 7.62,12.7
N$52  (via drill 1.02 pad 1.88)
  other vias: 10.16,12.7
N$53  (via drill 1.02 pad 1.88)
  other vias: 12.7,12.7
N$54  (via drill 1.02 pad 1.88)
  other vias: 15.24,12.7
N$55  (via drill 1.02 pad 1.88)
  other vias: 17.78,12.7
N$56  (via drill 1.02 pad 1.88)
  other vias: 20.32,12.7
N$57  (via drill 1.02 pad 1.88)
  other vias: 22.86,12.7
N$58  (via drill 1.02 pad 1.88)
  other vias: 25.4,12.7
N$59  (via drill 1.02 pad 1.88)
  other vias: 27.94,12.7
N$60  (via drill 1.02 pad 1.88)
  other vias: 30.48,12.7
N$61  (via drill 1.02 pad 1.88)
  other vias: 33.02,12.7
N$62  (via drill 1.02 pad 1.88)
  other vias: 35.56,12.7
N$63  (via drill 1.02 pad 1.88)
  other vias: 38.1,12.7
N$64  (via drill 1.02 pad 1.88)
  other vias: 40.64,12.7
N$65  (via drill 1.02 pad 1.88)
  other vias: 43.18,12.7
N$66  (via drill 1.02 pad 1.88)
  other vias: 45.72,12.7
N$67  (via drill 1.02 pad 1.88)
  other vias: 7.62,10.16
N$68  (via drill 1.02 pad 1.88)
  other vias: 10.16,10.16
N$69  (via drill 1.02 pad 1.88)
  other vias: 12.7,10.16
N$70  (via drill 1.02 pad 1.88)
  other vias: 15.24,10.16
N$71  (via drill 1.02 pad 1.88)
  other vias: 17.78,10.16
N$72  (via drill 1.02 pad 1.88)
  other vias: 20.32,10.16
N$73  (via drill 1.02 pad 1.88)
  other vias: 22.86,10.16
N$74  (via drill 1.02 pad 1.88)
  other vias: 25.4,10.16
N$75  (via drill 1.02 pad 1.88)
  other vias: 27.94,10.16
N$76  (via drill 1.02 pad 1.88)
  other vias: 30.48,10.16
N$77  (via drill 1.02 pad 1.88)
  other vias: 33.02,10.16
N$78  (via drill 1.02 pad 1.88)
  other vias: 35.56,10.16
N$79  (via drill 1.02 pad 1.88)
  other vias: 38.1,10.16
N$80  (via drill 1.02 pad 1.88)
  other vias: 40.64,10.16
N$81  (via drill 1.02 pad 1.88)
  other vias: 43.18,10.16
N$82  (via drill 1.02 pad 1.88)
  other vias: 45.72,10.16
N$83  (via drill 1.02 pad 1.88)
  other vias: 7.62,7.62
N$84  (via drill 1.02 pad 1.88)
  other vias: 10.16,7.62
N$85  (via drill 1.02 pad 1.88)
  other vias: 12.7,7.62
N$86  (via drill 1.02 pad 1.88)
  other vias: 15.24,7.62
N$87  (via drill 1.02 pad 1.88)
  other vias: 17.78,7.62
N$88  (via drill 1.02 pad 1.88)
  other vias: 20.32,7.62
N$89  (via drill 1.02 pad 1.88)
  other vias: 22.86,7.62
N$90  (via drill 1.02 pad 1.88)
  other vias: 25.4,7.62
N$91  (via drill 1.02 pad 1.88)
  other vias: 27.94,7.62
N$92  (via drill 1.02 pad 1.88)
  other vias: 30.48,7.62
N$93  (via drill 1.02 pad 1.88)
  other vias: 33.02,7.62
N$94  (via drill 1.02 pad 1.88)
  other vias: 35.56,7.62
N$95  (via drill 1.02 pad 1.88)
  other vias: 38.1,7.62
N$96  (via drill 1.02 pad 1.88)
  other vias: 40.64,7.62
N$97  (via drill 1.02 pad 1.88)
  other vias: 43.18,7.62
N$98  (via drill 1.02 pad 1.88)
  other vias: 45.72,7.62
N$99  (via drill 1.02 pad 1.88)
  other vias: 7.62,5.08
N$100  (via drill 1.02 pad 1.88)
  other vias: 10.16,5.08
N$101  (via drill 1.02 pad 1.88)
  other vias: 12.7,5.08
N$102  (via drill 1.02 pad 1.88)
  other vias: 15.24,5.08
N$103  (via drill 1.02 pad 1.88)
  other vias: 17.78,5.08
N$104  (via drill 1.02 pad 1.88)
  other vias: 20.32,5.08
N$105  (via drill 1.02 pad 1.88)
  other vias: 22.86,5.08
N$106  (via drill 1.02 pad 1.88)
  other vias: 25.4,5.08
N$107  (via drill 1.02 pad 1.88)
  other vias: 27.94,5.08
N$108  (via drill 1.02 pad 1.88)
  other vias: 30.48,5.08
N$109  (via drill 1.02 pad 1.88)
  other vias: 33.02,5.08
N$110  (via drill 1.02 pad 1.88)
  other vias: 35.56,5.08
N$111  (via drill 1.02 pad 1.88)
  other vias: 38.1,5.08
N$112  (via drill 1.02 pad 1.88)
  other vias: 40.64,5.08
N$113  (via drill 1.02 pad 1.88)
  other vias: 43.18,5.08
N$114  (via drill 1.02 pad 1.88)
  other vias: 45.72,5.08
N$115  (via drill 1.02 pad 1.88)
  other vias: 10.16,2.54
N$116  (via drill 1.02 pad 1.88)
  other vias: 12.7,2.54
N$117  (via drill 1.02 pad 1.88)
  other vias: 15.24,2.54
N$118  (via drill 1.02 pad 1.88)
  other vias: 17.78,2.54
N$119  (via drill 1.02 pad 1.88)
  other vias: 20.32,2.54
N$120  (via drill 1.02 pad 1.88)
  other vias: 22.86,2.54
N$121  (via drill 1.02 pad 1.88)
  other vias: 25.4,2.54
N$122  (via drill 1.02 pad 1.88)
  other vias: 27.94,2.54
N$123  (via drill 1.02 pad 1.88)
  other vias: 30.48,2.54
N$124  (via drill 1.02 pad 1.88)
  other vias: 33.02,2.54
N$125  (via drill 1.02 pad 1.88)
  other vias: 35.56,2.54
N$126  (via drill 1.02 pad 1.88)
  other vias: 38.1,2.54
N$127  (via drill 1.02 pad 1.88)
  other vias: 40.64,2.54
N$128  (via drill 1.02 pad 1.88)
  other vias: 43.18,2.54
N$129  (via drill 1.02 pad 1.88)
  other vias: 45.72,2.54
PICO
  Top 0.203: U3.7 19.68,25.91 19.43,26.16 3.3,26.16 U1.D11
PICO-IN  (via drill 0.38)
  Top 0.203: v41.91,39.37 41.91,39.75 41.27,40.39 40.51,40.39 39.98,39.85 U5.16 | U3.6 v18.41,23.49
  Bottom 0.203: v41.91,39.37 41.91,38.35 39.37,35.81 27.94,35.81 18.41,26.29 v18.41,23.49
POCI  (via drill 0.38)
  Top 0.203: v41.03,39.75 v41.02,39.75 40.62,39.35 U5.15
  Bottom 0.203: v41.03,39.75 40.4,39.12 40.01,39.12 38.23,37.34 27.3,37.34 15.88,25.91 13.97,25.91 11.43,23.37 4.32,23.37 3.81,22.86 U1.D12
RESET
  Top 0.203: U3.9 20.95,32.13 20.57,32.51 18.67,32.51 17.65,31.5 11.3,31.5 | R4.1 11.3,31.5 | 11.3,31.5 11.3,30.48 10.79,29.97 7.49,29.97 6.1,31.37 6.1,33.27 U1.D7
RESET-IN  (via drill 0.38)
  Top 0.203: v42.16,37.46 40.47,37.46 40.09,37.85 U5.12 | U3.10 v19.68,31.88
  Bottom 0.203: v42.16,37.46 42.67,37.97 42.67,39.5 41.78,40.39 40.64,40.39 38.1,37.85 27.05,37.85 21.08,31.88 v19.68,31.88
SCK
  Top 0.203: U3.3 14.61,22.86 13.84,22.1 9.02,22.1 7.24,20.32 U1.D13
SCK-IN  (via drill 0.38)
  Top 0.203: v40.14,38.4 40.14,38.35 U5.13 | U3.2 v13.34,23.49
  Bottom 0.203: v40.14,38.4 38.57,36.83 27.56,36.83 16.13,25.4 14.35,25.4 13.34,24.38 v13.34,23.49
VBCOMP
  Top 0.203: U5.22 34.81,44.12 C3.1
VBUS
  Top 0.254: J1.VBUS1 37.88,54.24 37.16,54.97 33.96,54.97 32.98,53.99 J1.VBUS2 33.02,53.64 33.02,52.84 31.12,50.93 F1.1
VDD  (via drill 0.38)
  Top 0.203: R9.2 v39.37,48.26 | v33.66,48.26 R10.2
  Top 0.254: v33.66,48.26 27.05,48.26 24.13,51.18 D2.A 19.43,53.98 | U6.3 6.67,41.59 6.99,41.91 8.51,41.91 8.57,41.85 | U6.1 8.57,41.85 | 8.57,41.85 8.57,52.89 12.06,56.39 18.54,56.39 19.43,55.5 19.43,53.98 | S1.1 18.89,49.63 19.43,50.16 19.43,53.98
  Bottom 0.254: v33.66,48.26 v39.37,48.26
VIN  (via drill 0.38)
  Top 0.254: C1.1 10.29,33.44 C6.+ 10.29,36.83 11.43,37.97 11.43,38.73 11.86,39.17 U2.3 12.93,40.49 13.21,40.77 13.59,40.77 v13.97,41.15
  Bottom 0.254: v13.97,41.15 45.97,41.15 47.62,39.5 47.62,39.12 48.9,37.85 49.78,37.85 U1.VIN
XI
  Top 0.203: Y1.P3 31.39,42.67 32.51,42.67 | 32.51,42.67 33.53,42.67 33.81,42.39 U5.24 | C10.1 30.86,44.2 31.5,43.56 32.13,43.56 32.51,43.18 32.51,42.67
XO
  Top 0.203: 29.63,39.85 Y1.P1 | 29.63,39.85 28.18,39.85 C9.1 | U5.25 29.63,39.85

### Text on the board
Bottom: V01
tDocu: A. Weiss | M. Chodikov

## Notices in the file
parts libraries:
SparkFun-Aesthetics: Licensing: Creative Commons ShareAlike 4.0 International - https://creativecommons.org/licenses/by-sa/4.0
SparkFun-Aesthetics: Released under the Creative Commons Attribution Share-Alike 4.0 License
SparkFun-Aesthetics: https://creativecommons.org/licenses/by-sa/4.0
